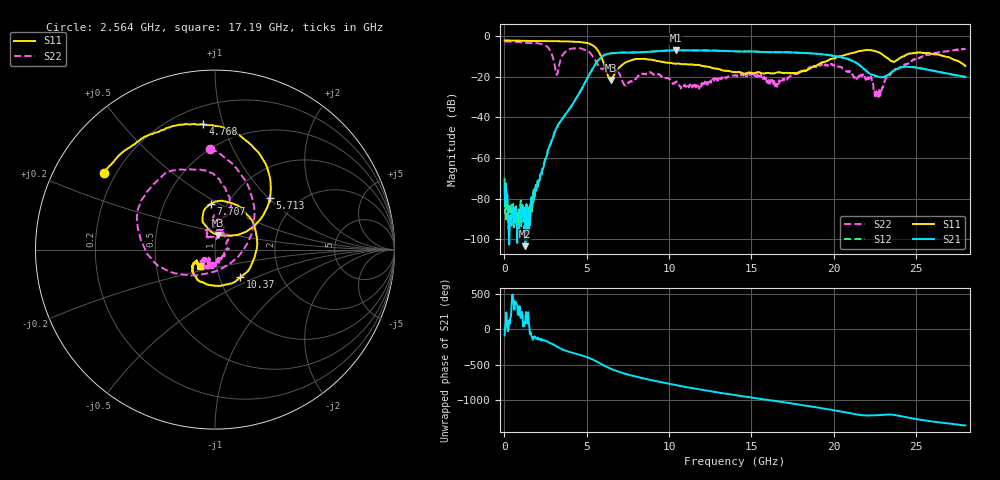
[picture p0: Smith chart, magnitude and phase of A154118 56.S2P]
!  2-Port S-parameters saved by WinCal
! VAR MeasName=S-Parameters (CALIBRATED_DATA) read from VNA (N5230A)
! VAR MeasDate=2015-9-10 14:39:26
! VAR NAME=A154118 56
! VAR FILENAME=A154118 56.S2P
! VAR DATE=2015-9-10 14:39:26
! VAR PHYS_PORTS=1,2
# Hz S DB R 50
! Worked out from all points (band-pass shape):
!   801 points, 10 MHz to 28 GHz, reference 50 ohm
!   highest |S21| = -6.96 dB at 10.44 GHz (marker M1); lowest = -103.3 dB at 1.27 GHz (marker M2)
!   |S21| within 3 dB of the highest: 5.946 GHz to 20.18 GHz (14.23 GHz wide, 109 % of centre)
!   lowest |S11| = -21.6 dB at 6.448 GHz (marker M3), VSWR 1.18, Z = 50.7 + j8.4 ohm
!   |S11| at or under -10 dB: 5.872 GHz to 20.33 GHz (14.46 GHz wide, 110 % of centre); 23.12 GHz to 24.22 GHz (1.099 GHz wide, 4.65 % of centre); 26.73 GHz to end of sweep
!   |S22| runs from -30.1 to -2.7 dB; largest |S21 - S12| = 0.0078
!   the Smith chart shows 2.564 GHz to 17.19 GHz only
!   S11 on the Smith chart (normalised r, x): 2.564 GHz: 0.15, +0.31; 4.768 GHz: 0.31, +0.86; 5.713 GHz: 1.46, +1.02; 7.707 GHz: 0.84, +0.45; 10.37 GHz: 1.25, -0.41; 17.19 GHz: 0.83, -0.16
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1e7  -2.15 179.7  -73.41 -84.7  -69.76 -99.2  -2.68 179.8
1.26955e9  -2.34 163.1  -103.35 96.3  -96.41 -149.1  -3.34 149.2
1.724388e9  -2.41 157.3  -80.57 -146.4  -82.03 -81.1  -3.44 137.7
2.564088e9  -2.46 145.3  -59.22 -168.0  -59.24 -167.1  -5.00 92.8
2.94895e9  -2.53 139.2  -50.02 152.4  -50.04 152.1  -10.71 40.9
3.333812e9  -2.53 132.5  -42.67 99.3  -42.64 99.5  -13.96 -134.0
3.858625e9  -2.60 121.8  -36.91 49.6  -36.94 49.5  -6.82 161.2
4.698325e9  -3.05 98.2  -25.91 -5.8  -25.87 -6.0  -6.22 114.0
4.7683e9  -3.09 95.5  -24.81 -11.0  -24.78 -10.9  -6.49 110.3
5.712962e9  -7.56 43.3  -11.71 -105.9  -11.67 -105.8  -14.37 74.0
6.4477e9  -21.57 80.2  -8.51 167.7  -8.45 167.6  -14.60 87.3
7.70725e9  -11.91 95.6  -8.13 71.7  -8.09 71.5  -22.08 119.0
9.351662e9  -12.32 15.3  -7.42 -14.7  -7.35 -14.8  -18.70 70.5
1.03663e10  -13.60 -47.8  -7.00 -62.3  -6.95 -62.6  -22.63 3.6
1.043628e10  -13.54 -52.8  -6.96 -65.4  -6.93 -65.8  -22.55 0.6
1.4005e10  -17.77 -148.6  -7.52 155.6  -7.49 155.2  -19.37 -115.9
1.718886e10  -18.19 -131.9  -7.97 47.3  -7.90 46.5  -20.94 -107.3
1.869332e10  -15.25 -107.7  -8.52 -6.9  -8.54 -7.3  -14.63 -106.2
2.219208e10  -6.92 -154.1  -18.51 -130.5  -18.41 -131.6  -19.62 -177.1
2.257694e10  -7.46 -165.8  -19.69 -127.7  -19.65 -129.1  -27.03 120.0
2.334666e10  -11.43 -173.2  -18.81 -116.3  -18.77 -117.9  -18.89 -11.7
2.8e10  -14.76 139.2  -20.03 88.6  -20.12 87.6  -6.08 -101.3
